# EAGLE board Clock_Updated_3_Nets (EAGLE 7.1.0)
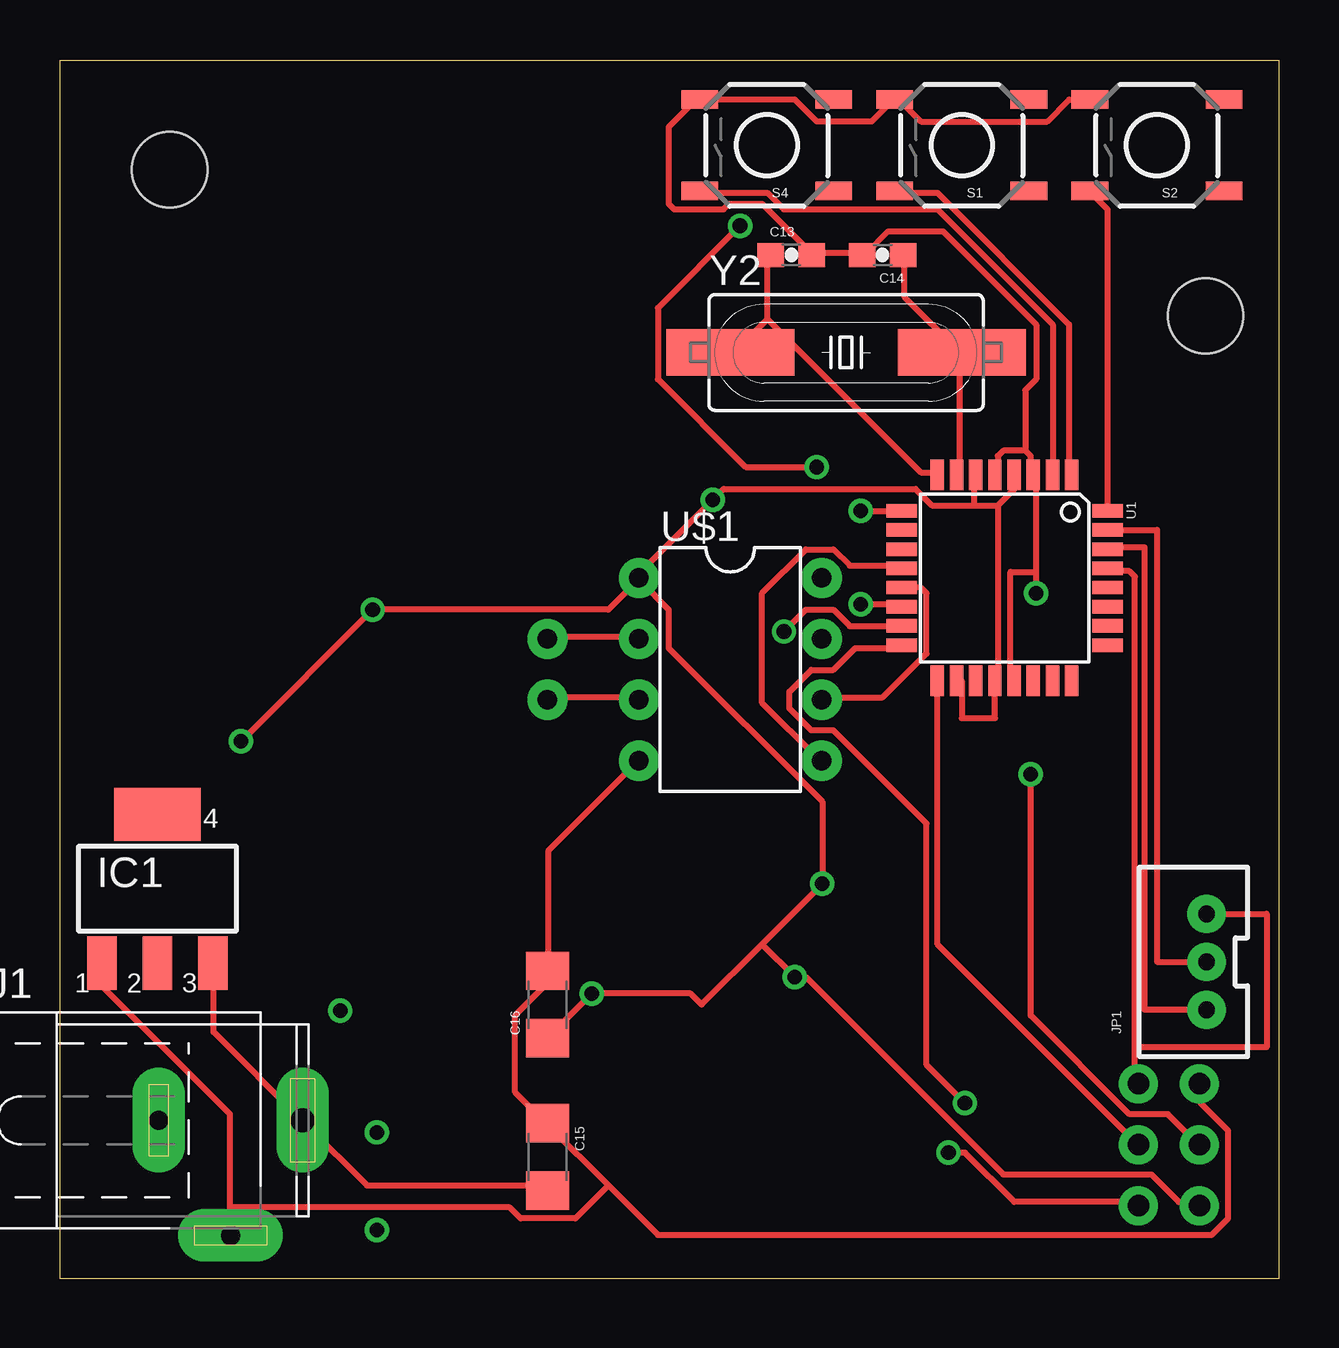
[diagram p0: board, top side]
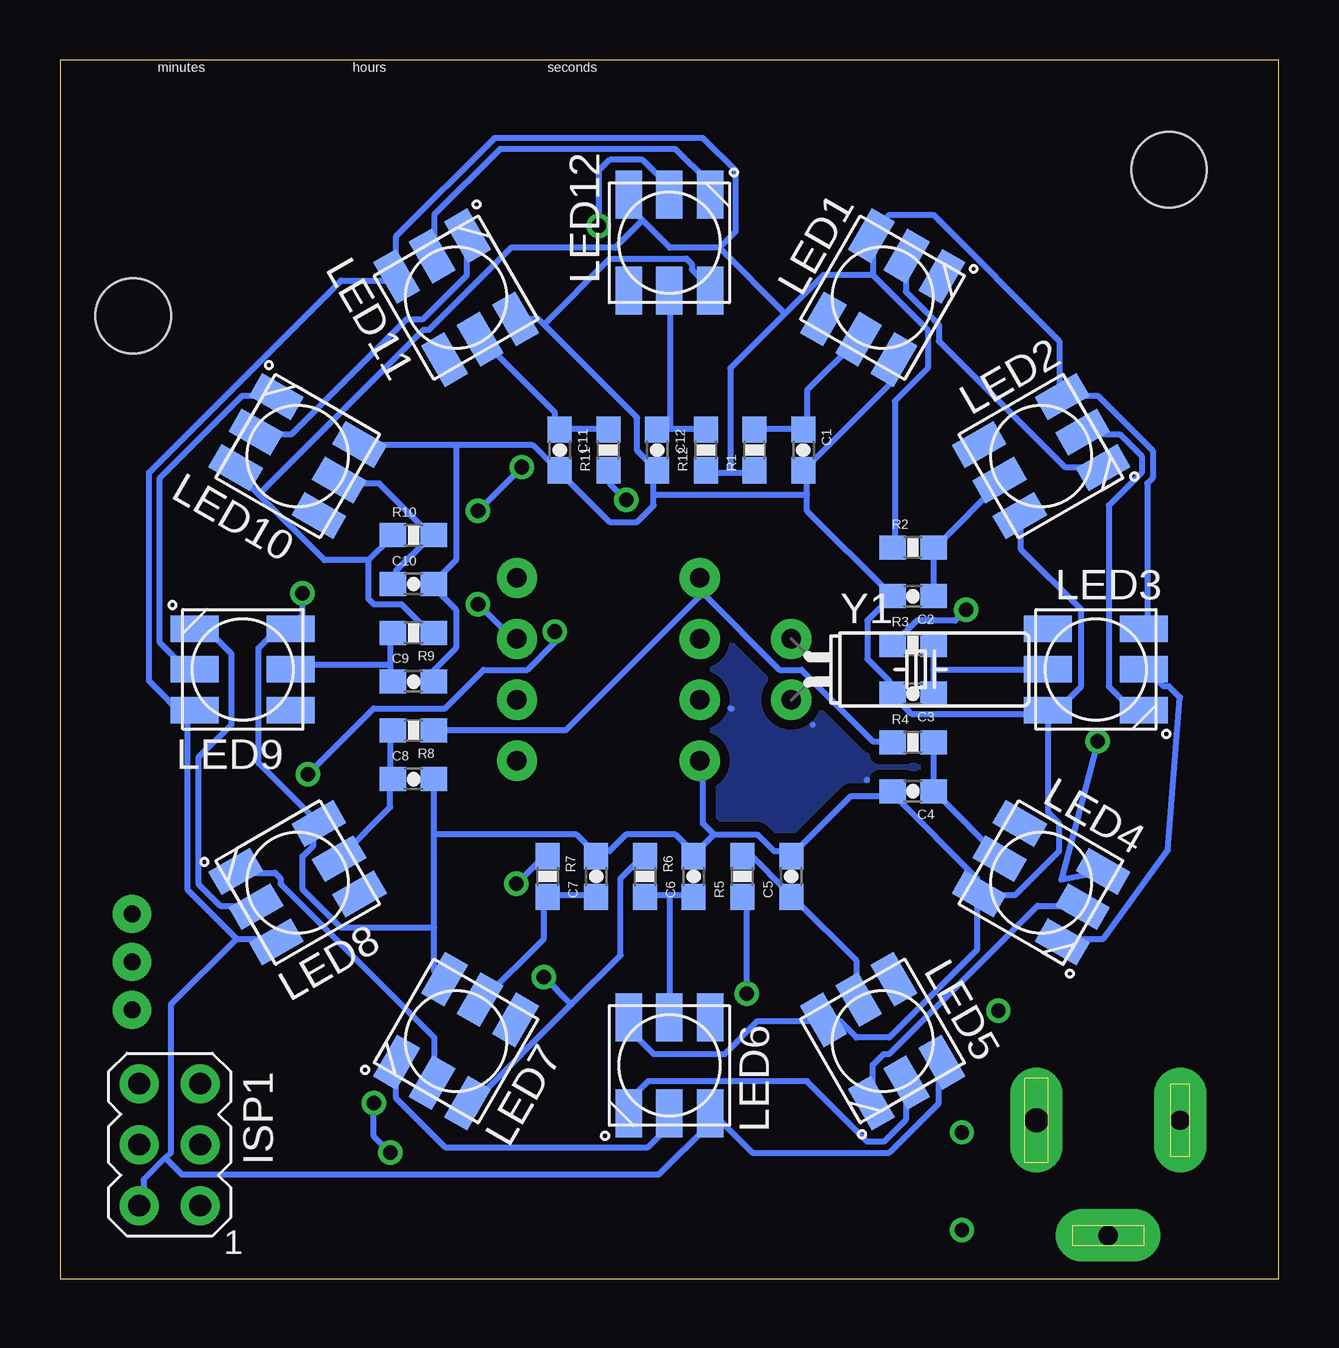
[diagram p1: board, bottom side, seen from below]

Size 50.8 x 50.8 mm. Coordinates in mm from the lower left corner, seen from the top.
Outline: 50.8,0 0,0 0,50.8 50.8,50.8 50.8,0
Copper layers (1*16): Top 0.035mm / dielectric 1.5mm / Bottom 0.035mm
Design rules "default": minimum track width 10mil, minimum drill 24mil, track to track 8mil, track to pad 8mil, pad to pad 8mil, via to via 8mil, smd to smd 8mil, copper to edge 40mil, drill to drill 8mil, minimum pad ring 10mil, minimum via ring 8mil, stop-mask expansion 4mil, vias tented up to drill 0mil, thermal gap 10mil
Holes 3.14 mm at 4.57,46.23 47.75,40.13

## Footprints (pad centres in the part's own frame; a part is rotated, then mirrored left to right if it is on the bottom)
0603-CAP = smd 1.1 x 1: 1 -0.85,0; 2 0.85,0
1206 = smd 1.6 x 1.8: 1 -1.4,0; 2 1.4,0
SOT223 = smd 1.219 x 2.235: 1 -2.311,-3.099; 2 0,-3.099; 3 2.311,-3.099 | smd 3.6 x 2.2: 4 0,3.099
AVRISP = drill 0.9 pad 1.626: 1 -1.27,2.54; 2 1.27,2.54; 3 -1.27,0; 4 1.27,0; 5 -1.27,-2.54; 6 1.27,-2.54
SPC4077 = drill 0.8 pad 2.184 long: 1 -3,0; 2 0,-4.8 | drill 1 pad 2.184 long: 3 3,0
JST-3-PTH-VERT = drill 0.7 pad 1.6: 1 -2,-0.55; 2 0,-0.55; 3 2,-0.55
WS2812 = smd 2 x 1.1: DI 2,0; DO 2,-1.7; LEDVDD -2,0; NC -2,1.7; VDD 2,1.7; VSS -2,-1.7
0603-RES = smd 1.1 x 1: 1 -0.85,0; 2 0.85,0
TACTILE-SWITCH-SMD = smd 1.524 x 0.762: 1 -2.794,1.905; 2 2.794,1.905; 3 -2.794,-1.905; 4 2.794,-1.905
TQFP32-08 = smd 1.27 x 0.559: 1 -4.293,2.8; 2 -4.293,2; 3 -4.293,1.2; 4 -4.293,0.4; 5 -4.293,-0.4; 6 -4.293,-1.2; 7 -4.293,-2; 8 -4.293,-2.8; 17 4.293,-2.8; 18 4.293,-2; 19 4.293,-1.2; 20 4.293,-0.4; 21 4.293,0.4; 22 4.293,1.2; 23 4.293,2; 24 4.293,2.8 | smd 0.559 x 1.27: 9 -2.8,-4.293; 10 -2,-4.293; 11 -1.2,-4.293; 12 -0.4,-4.293; 13 0.4,-4.293; 14 1.2,-4.293; 15 2,-4.293; 16 2.8,-4.293; 25 2.8,4.293; 26 2,4.293; 27 1.2,4.293; 28 0.4,4.293; 29 -0.4,4.293; 30 -1.2,4.293; 31 -2,4.293; 32 -2.8,4.293
DIL08-ROUND = drill 0.813 pad 1.676: 1 -3.81,-3.81; 2 -1.27,-3.81; 3 1.27,-3.81; 4 3.81,-3.81; 5 3.81,3.81; 6 1.27,3.81; 7 -1.27,3.81; 8 -3.81,3.81
TC38H = drill 0.813 pad 1.676: 1 -1.27,0; 2 1.27,0
HC49UP = smd 5.334 x 1.93: 1 -4.826,0; 2 4.826,0

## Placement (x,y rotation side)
C1  0.1uF  [0603-CAP]  19.81,34.54 270 bottom
C2  0.1uF  [0603-CAP]  15.24,28.45 180 bottom
C3  0.1uF  [0603-CAP]  15.24,24.38 180 bottom
C4  0.1uF  [0603-CAP]  15.24,20.32 180 bottom
C5  0.1uF  [0603-CAP]  20.32,16.76 90 bottom
C6  0.1uF  [0603-CAP]  24.38,16.76 90 bottom
C7  0.1uF  [0603-CAP]  28.45,16.76 90 bottom
C8  0.1uF  [0603-CAP]  36.07,20.83 0 bottom
C9  0.1uF  [0603-CAP]  36.07,24.89 0 bottom
C10  0.1uF  [0603-CAP]  36.07,28.96 0 bottom
C11  0.1uF  [0603-CAP]  29.97,34.54 270 bottom
C12  0.1uF  [0603-CAP]  25.91,34.54 270 bottom
C13  22pF  [0603-CAP]  30.48,42.67 0 top
C14  22pF  [0603-CAP]  34.29,42.67 180 top
C15  10uF  [1206]  20.32,5.08 270 top
C16  10uF  [1206]  20.32,11.43 90 top
IC1  317EMP  [SOT223]  4.06,16.26 0 top
ISP1  AVRISP-6  [AVRISP]  46.23,5.59 180 bottom
J1  [SPC4077]  7.11,6.6 0 top
JP1  [JST-3-PTH-VERT]  47.24,13.21 90 top
LED1  WS2812  [WS2812]  16.51,40.89 60 bottom
LED2  WS2812  [WS2812]  9.91,34.29 30 bottom
LED3  WS2812  [WS2812]  7.62,25.4 0 bottom
LED4  WS2812  [WS2812]  9.91,16.51 330 bottom
LED5  WS2812  [WS2812]  16.51,9.91 300 bottom
LED6  WS2812  [WS2812]  25.4,8.89 270 bottom
LED7  WS2812  [WS2812]  34.29,9.91 240 bottom
LED8  WS2812  [WS2812]  40.89,16.51 210 bottom
LED9  WS2812  [WS2812]  43.18,25.4 180 bottom
LED10  WS2812  [WS2812]  40.89,34.29 150 bottom
LED11  WS2812  [WS2812]  34.29,40.89 120 bottom
LED12  WS2812  [WS2812]  25.4,43.18 90 bottom
R1  180  [0603-RES]  21.84,34.54 90 bottom
R2  180  [0603-RES]  15.24,30.48 0 bottom
R3  180  [0603-RES]  15.24,26.42 0 bottom
R4  180  [0603-RES]  15.24,22.35 0 bottom
R5  180  [0603-RES]  22.35,16.76 90 bottom
R6  180  [0603-RES]  26.42,16.76 270 bottom
R7  180  [0603-RES]  30.48,16.76 270 bottom
R8  180  [0603-RES]  36.07,22.86 180 bottom
R9  180  [0603-RES]  36.07,26.92 180 bottom
R10  180  [0603-RES]  36.07,30.99 0 bottom
R11  180  [0603-RES]  27.94,34.54 90 bottom
R12  180  [0603-RES]  23.88,34.54 90 bottom
S1  TAC_SWITCHSMD  [TACTILE-SWITCH-SMD]  37.59,47.24 180 top
S2  TAC_SWITCHSMD  [TACTILE-SWITCH-SMD]  45.72,47.24 180 top
S4  TAC_SWITCHSMD  [TACTILE-SWITCH-SMD]  29.46,47.24 180 top
U1  ATMEGA328P  [TQFP32-08]  39.37,29.21 270 top
U$1  DS1302  [DIL08-ROUND]  27.94,25.4 270 top
Y1  [TC38H]  20.32,25.4 270 bottom
Y2  [HC49UP]  32.77,38.61 0 top

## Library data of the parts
C1-C12 = SparkFun-Capacitors; PROD_ID: CAP-00810
C13 C14 = SparkFun-Capacitors; PROD_ID: CAP-07876
C15 C16 = SparkFun-Capacitors; PROD_ID: CAP-10057
IC1 = linear
ISP1 LED1-LED12 U$1 = adafruit
J1 = con-jack; OC_FARNELL: unknown; OC_NEWARK: unknown
JP1 = SparkFun-Connectors
R1-R12 = SparkFun-Resistors; PROD_ID: RES-08788
S1 S2 S4 = SparkFun-Electromechanical; PROD_ID: SWCH-08247
U1 = SparkFun-DigitalIC; PROD_ID: IC-09069
Y1 Y2 = SparkFun-FreqCtrl

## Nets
GND: C1.2 C2.2 C3.2 C4.2 C5.2 C6.2 C7.2 C8.2 C9.2 C10.2 C11.2 C12.2 C13.2 C14.2 C15.1 C16.2 IC1.1 ISP1.6 J1.2 LED1.VSS LED2.VSS LED3.VSS LED4.VSS LED5.VSS LED6.VSS LED7.VSS LED8.VSS LED9.VSS LED10.VSS LED11.VSS LED12.VSS S1.4 S2.4 S4.4 U1.3 U1.5 U1.21 U$1.4
N$1: ISP1.4 U1.15
N$2: ISP1.1 U1.16
N$3: JP1.1 U1.30
N$4: S2.2 U1.32
N$5: U$1.3 Y1.2
N$6: U$1.2 Y1.1
N$7: C1.1 LED1.LEDVDD R1.2
N$8: C2.1 LED2.LEDVDD R2.2
N$9: LED1.DI LED2.DO
N$10: C3.1 LED3.LEDVDD R3.2
N$11: C4.1 LED4.LEDVDD R4.2
N$12: LED3.DI LED4.DO
N$13: C5.1 LED5.LEDVDD R5.2
N$14: C6.1 LED6.LEDVDD R6.2
N$15: LED5.DI LED6.DO
N$16: C7.1 LED7.LEDVDD R7.2
N$17: C8.1 LED8.LEDVDD R8.2
N$18: LED7.DI LED8.DO
N$19: C9.1 LED9.LEDVDD R9.2
N$20: C10.1 LED10.LEDVDD R10.2
N$21: LED9.DI LED10.DO
N$22: C11.1 LED11.LEDVDD R11.2
N$23: C12.1 LED12.LEDVDD R12.2
N$24: LED11.DI LED12.DO
N$25: LED4.DI LED5.DO
N$26: LED8.DI LED9.DO
N$27: JP1.2 U1.31
N$30: S1.2 U1.1
N$31: U1.13 U$1.6
N$32: U1.12 U$1.5
N$33: U1.14 U$1.7
N$34: ISP1.3 U1.17
N$36: ISP1.5 JP1.3 U1.29
N$37: S4.2 U1.2
N$38: C13.1 U1.8 Y2.1
N$40: LED2.DI LED3.DO
N$41: LED6.DI LED7.DO
N$42: LED10.DI LED11.DO
N$43: LED12.DI U1.9
N$44: C14.1 U1.7 Y2.2
N$45: C15.2 IC1.3 J1.3
VBAT: U$1.8
VCC: C16.1 ISP1.2 LED1.VDD LED2.VDD LED3.VDD LED4.VDD LED5.VDD LED6.VDD LED7.VDD LED8.VDD LED9.VDD LED10.VDD LED11.VDD LED12.VDD R1.1 R2.1 R3.1 R4.1 R5.1 R6.1 R7.1 R8.1 R9.1 R10.1 R11.1 R12.1 U1.4 U1.6 U1.18 U1.20 U$1.1

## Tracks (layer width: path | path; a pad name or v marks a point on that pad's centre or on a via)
GND  (via drill 0.61)
  Top 0.254: 40.23,34.52 39.32,34.52 39.09,34.29 39.09,33.6 U1.5 | 40.23,34.52 40.46,34.29 40.46,33.6 U1.3 40.69,33.38 40.69,29.46 | S2.4 42.06,49.15 41.15,48.23 35.89,48.23 34.98,49.15 S1.4 34.75,49.15 33.83,48.23 31.55,48.23 30.63,49.15 S4.4 26.52,49.15 25.38,48.01 25.38,44.81 25.6,44.58 27.66,44.58 27.89,44.81 29.26,44.81 31.32,42.75 C13.2 31.55,42.75 33.38,42.75 C14.2 33.6,42.75 34.52,43.66 36.8,43.66 40.69,39.78 40.69,37.49 40.23,37.03 40.23,34.52 | v40.69,28.57 40.69,29.46 | U$1.4 24,21.49 20.34,17.83 20.34,13.03 C16.2 20.12,12.8 20.12,12.12 18.97,10.97 18.97,7.77 20.12,6.63 C15.1 20.34,6.4 22.86,3.89 | U1.21 39.62,24.92 39.62,29.46 40.69,29.46 | 7.09,2.97 7.09,1.83 J1.2 | 7.09,2.97 7.09,6.86 1.83,12.12 1.83,13.03 IC1.1 | 22.86,3.89 24.92,1.83 48.01,1.83 48.69,2.52 48.69,6.17 47.55,7.32 47.55,8 ISP1.6 | 7.09,2.97 18.75,2.97 19.2,2.52 21.49,2.52 22.86,3.89
  Bottom 0.254: LED1.VSS 16.23,38.18 16.23,37.26 19.66,33.83 C1.2 19.66,33.6 19.66,32.69 | LED3.VSS 9.83,23.55 15.32,23.55 16,24.23 C3.2 16.23,24.46 16.23,24.92 17.14,25.83 17.14,27.43 16.23,28.35 C2.2 16.23,28.57 19.66,32 19.66,32.69 | LED2.VSS 10.74,31.77 10.74,30.4 8.23,27.89 8.23,24.69 9.14,23.77 9.6,23.77 LED3.VSS | C9.2 35.2,24.92 35.2,25.38 34.29,26.29 34.29,27.89 35.2,28.8 C10.2 35.2,29.03 34.29,29.95 34.29,34.75 | 26.06,32.69 26.06,32.23 26.75,31.55 27.89,31.55 29.95,33.6 C11.2 30.18,33.83 31.09,34.75 34.29,34.75 | 26.06,32.69 26.06,33.6 C12.2 26.06,33.83 26.75,34.52 26.75,35.89 30.63,39.78 | 34.29,34.75 38.18,34.75 LED10.VSS | 30.63,39.78 30.86,40.01 31.77,40.01 LED11.VSS | 30.63,39.78 27.89,42.52 24.69,42.52 24.46,42.29 24.46,42.06 23.77,41.38 LED12.VSS | 26.06,32.69 19.66,32.69 | 35.2,14.63 35.2,12.8 34.98,12.57 LED7.VSS | 35.2,14.63 35.2,18.52 | 35.2,18.52 35.2,20.8 C8.2 | 35.2,14.63 39.09,14.63 40.69,16.23 40.69,17.6 40.23,18.06 40.23,18.97 LED8.VSS 40.23,19.2 42.52,21.49 42.52,26.29 41.83,26.98 41.38,26.98 LED9.VSS 41.15,27.2 40.69,27.66 v40.69,28.57 | LED6.VSS 26.98,10.74 26.98,10.29 26.06,9.37 23.09,9.37 21.72,10.74 19.2,10.74 LED5.VSS 18.97,10.74 18.29,10.74 17.6,10.06 16.23,10.06 12.57,13.72 12.57,16 LED4.VSS | 23.55,18.52 21.72,18.52 21.03,17.83 20.34,17.83 C5.2 20.12,17.83 17.83,20.12 16.23,20.12 C4.2 16,20.12 12.57,16.69 12.57,16.23 LED4.VSS | 23.55,18.52 24.23,17.83 C6.2 24.46,17.83 25.15,18.52 27.2,18.52 27.89,17.83 28.35,17.83 C7.2 28.57,17.83 29.26,18.52 35.2,18.52 | 23.55,18.52 24,18.97 24,21.49 U$1.4 | LED3.VSS 9.6,23.55 9.6,19.43 9.14,18.97 9.14,17.83 10.97,16 12.34,16 LED4.VSS
N$1  (via drill 0.61)
  Top 0.254: v30.18,26.98 31.09,27.89 32.23,27.89 32.92,27.2 34.98,27.2 U1.15 | v40.46,21.03 40.46,10.97 44.58,6.86 46.18,6.86 47.32,5.71 ISP1.4
  Bottom 0.254: v30.18,26.98 30.18,26.52 31.32,25.38 33.15,25.38 34.75,23.77 37.72,23.77 v40.46,21.03
N$2  (via drill 0.61)
  Top 0.254: v37.72,7.32 36.12,8.91 36.12,18.97 32.23,22.86 31.32,22.86 30.4,23.77 30.4,24.46 31.32,25.38 32.23,25.38 33.15,26.29 34.98,26.29 U1.16 | v37.03,5.26 37.72,5.26 39.78,3.2 44.81,3.2 ISP1.1
  Bottom 0.254: v37.72,7.32 37.72,5.94 v37.03,5.26
N$3
  Top 0.254: JP1.1 45.21,11.21 45.21,30.48 43.66,30.48 U1.30
N$4
  Top 0.254: U1.32 43.66,44.58 42.98,45.26 S2.2
N$5
  Top 0.254: Y1.2 20.34,24.23 24,24.23 U$1.3
N$6
  Top 0.254: Y1.1 20.34,26.75 24,26.75 U$1.2
N$7
  Bottom 0.254: R1.2 21.72,35.43 19.89,35.43 C1.1 19.66,35.43 19.66,37.03 17.6,39.09 LED1.LEDVDD
N$8
  Bottom 0.254: C2.1 14.4,28.57 14.4,30.4 R2.2 14.17,30.63 11.66,33.15 LED2.LEDVDD
N$9
  Bottom 0.254: LED2.DO 7.54,33.83 8.91,33.83 14.17,39.09 14.17,39.78 15.54,41.15 15.54,42.52 LED1.DI
N$10
  Bottom 0.254: 14.4,25.38 14.4,26.29 R3.2 | 14.4,25.38 14.4,24.46 C3.1 | 14.4,25.38 9.83,25.38 LED3.LEDVDD
N$11
  Bottom 0.254: R4.2 14.4,22.17 14.4,20.34 C4.1 14.17,20.12 11.66,17.6 LED4.LEDVDD
N$12
  Bottom 0.254: LED3.DI 5.49,25.38 4.8,24.69 4.57,24.69 4.12,24.23 4.62,17.88 7.32,14.17 8.91,14.17 LED4.DO
N$13
  Bottom 0.254: R5.2 22.17,17.83 20.34,16 C5.1 20.12,15.77 17.6,13.26 17.6,11.66 LED5.LEDVDD
N$14
  Bottom 0.254: 25.38,16 26.29,16 R6.2 | 25.38,16 24.46,16 C6.1 | 25.38,16 25.38,10.97 LED6.LEDVDD
N$15
  Bottom 0.254: LED6.DO 26.98,7.09 26.98,7.54 26.29,8.23 19.66,8.23 17.14,5.71 16.46,5.71 15.54,6.63 15.54,8 LED5.DI
N$16
  Bottom 0.254: C7.1 28.57,16 30.4,16 R7.2 30.63,15.77 30.63,14.17 33.15,11.66 LED7.LEDVDD
N$17
  Bottom 0.254: R8.2 37.03,22.86 37.03,21.03 C8.1 37.03,20.8 37.03,19.66 39.09,17.6 LED8.LEDVDD
N$18
  Bottom 0.254: LED7.DI 35.2,8.23 35.2,10.06 41.6,16.46 41.6,16.69 41.83,16.92 43.43,16.92 LED8.DO
N$19
  Bottom 0.254: 37.03,25.6 37.03,26.75 R9.2 | 37.03,25.6 37.03,24.92 C9.1 | 37.03,25.6 41.15,25.6 LED9.LEDVDD
N$20
  Bottom 0.254: C10.1 36.8,29.03 36.8,29.49 35.43,30.86 R10.2 35.43,31.09 37.49,33.15 39.09,33.15 LED10.LEDVDD
N$21
  Bottom 0.254: LED10.DO 41.83,36.8 43.2,36.8 46.63,33.38 46.63,26.52 45.72,25.6 45.26,25.6 LED9.DI
N$22
  Bottom 0.254: R11.2 28.12,35.43 29.95,35.43 C11.1 30.18,35.43 30.18,36.12 33.15,39.09 LED11.LEDVDD
N$23
  Bottom 0.254: 25.38,35.43 25.83,35.43 C12.1 | 25.38,35.43 24,35.43 R12.2 | 25.38,35.43 25.38,41.15 LED12.LEDVDD
N$24
  Bottom 0.254: LED11.DI 35.2,42.75 35.2,44.35 32.46,47.09 25.15,47.09 23.77,45.72 23.77,45.26 LED12.DO
N$25
  Bottom 0.254: LED5.DO 16.92,7.54 16.92,8.91 16.46,9.37 16.23,9.37 10.06,15.54 8.23,15.54 LED4.DI
N$26
  Bottom 0.254: LED8.DI 42.75,15.54 44.12,15.54 45.03,16.46 45.03,21.72 43.66,23.09 43.66,26.06 44.58,26.98 45.03,26.98 LED9.DO
N$27
  Top 0.254: U1.31 45.72,31.21 45.72,13.21 JP1.2
N$28
  Bottom 0.254: 22.86,23.77 22.8,23.75 | 17.14,20.8 17.17,20.78 | 19.43,23.09 19.43,23.08
  pour Bottom (isolate 0.406): 0.51,50.29 50.29,50.29 50.8,50.29 50.8,0 0,0 0,50.29
N$29  (via drill 0.6)
  other vias: 13.21,2.03
N$30
  Top 0.254: U1.1 42.06,33.6 42.06,39.78 36.58,45.26 34.98,45.26 S1.2
N$31
  Top 0.254: U1.13 35.2,28.8 35.89,28.8 36.12,28.57 36.12,26.06 34.29,24.23 31.77,24.23 U$1.6
N$32
  Top 0.254: U1.12 34.98,29.72 32.92,29.72 32.23,30.4 31.09,30.4 29.26,28.57 29.26,24 31.55,21.72 U$1.5
N$33  (via drill 0.61)
  Top 0.254: v33.38,28.12 34.98,28.12 U1.14
  Bottom 0.254: v33.38,28.12 31.77,26.52 U$1.7
N$34
  Top 0.254: U1.17 36.58,13.95 44.81,5.71 ISP1.3
N$35  (via drill 0.6)
  other vias: 13.21,6.1
N$36
  Top 0.254: 44.81,9.65 44.81,8.23 ISP1.5 | 44.81,9.65 44.81,29.26 44.58,29.49 43.66,29.49 U1.29 | JP1.3 50.29,15.21 50.29,9.65 44.81,9.65
N$37
  Top 0.254: U1.2 41.38,33.6 41.38,39.78 36.58,44.58 30.18,44.58 29.49,45.26 26.75,45.26 S4.2
N$38
  Top 0.254: 29.49,40.01 29.49,42.52 C13.1 | 29.49,40.01 28.12,38.63 Y2.1 | 29.49,40.01 35.89,33.6 36.35,33.6 U1.8
N$39  (via drill 0.6)
  other vias: 11.68,11.18
N$40
  Bottom 0.254: LED3.DO 5.71,23.77 6.17,23.77 7.09,24.69 7.09,32.23 5.71,33.6 5.71,34.29 6.63,35.2 8,35.2 LED2.DI
N$41
  Bottom 0.254: LED6.DI 25.6,6.86 25.6,6.17 26.29,5.49 34.75,5.49 36.8,7.54 36.8,8.91 LED7.DO
N$42
  Bottom 0.254: LED11.DO 33.83,43.43 33.83,41.83 35.66,40.01 36.35,40.01 41.15,35.2 42.52,35.2 LED10.DI
N$43  (via drill 0.61)
  Top 0.254: v33.38,32 34.98,32 U1.9 | v31.55,33.83 28.57,33.83 24.92,37.49 24.92,40.46 v28.35,43.89
  Bottom 0.254: v31.55,33.83 v33.38,32 | v28.35,43.89 28.35,46.18 27.89,46.63 26.52,46.63 25.6,45.72 25.6,45.26 LED12.DI
N$44
  Top 0.254: C14.1 35.2,42.52 35.2,40.92 37.49,38.63 Y2.2 37.49,38.41 37.49,33.6 U1.7
N$45
  Top 0.254: C15.2 20.12,3.89 12.8,3.89 10.29,6.4 J1.3 10.06,6.63 6.4,10.29 6.4,13.03 IC1.3
VCC  (via drill 0.61)
  Top 0.254: C16.1 20.34,10.06 v22.17,11.89 26.29,11.89 26.75,11.43 29.26,13.95 | 29.26,13.95 v31.77,16.46 31.77,19.89 25.38,26.29 25.38,27.89 24.23,29.03 U$1.1 | 29.26,13.95 v30.63,12.57 31.09,12.57 39.32,4.34 45.49,4.34 46.63,3.2 47.32,3.2 ISP1.2 | 39.09,32.23 39.09,24.92 U1.20 38.97,23.37 37.59,23.37 37.59,24.92 U1.18 | 39.09,32.23 39.78,32.92 39.78,33.38 U1.4 | U$1.1 24,29.03 22.86,27.89 v13.03,27.89 v7.54,22.4 | U$1.1 24,29.26 v27.2,32.46 27.66,32.92 35.66,32.92 36.35,32.23 38.1,32.23 | 38.1,32.23 39.09,32.23 | U1.6 38.1,33.5 38.1,32.23
  Bottom 0.254: 37.95,29.95 37.95,28.35 37.72,28.12 36.58,28.12 35.43,26.98 R9.1 | 37.95,29.95 37.03,30.86 R10.1 | 42.52,32.69 39.78,29.95 37.95,29.95 | 42.52,32.69 43.43,33.6 LED10.VDD | LED3.VDD 5.49,27.2 5.49,33.15 5.26,33.38 5.26,34.52 7.54,36.8 8.91,36.8 LED2.VDD 9.14,36.8 9.14,39.09 14.4,44.35 16.23,44.35 16.92,43.66 LED1.VDD 16.92,43.43 16.92,41.83 | 22.86,33.6 23.77,33.6 R12.1 | 22.86,33.6 21.95,33.6 R1.1 | 16.92,41.83 14.63,39.55 14.63,37.95 16,36.58 16,30.63 R2.1 | 22.86,33.6 22.86,37.95 20.57,40.23 | 20.57,40.23 18.97,41.83 16.92,41.83 | 26.52,44.12 25.38,42.98 23.32,42.98 | 26.52,44.12 26.98,44.58 26.98,45.03 LED12.VDD | 20.57,40.23 23.32,42.98 | 23.32,42.98 22.63,43.66 22.63,46.18 24,47.55 32.69,47.55 36.8,43.43 36.8,41.83 LED11.VDD 36.8,41.6 39.09,41.6 47.09,33.6 47.09,24.92 45.49,23.32 | 42.52,32.69 35.66,39.55 35.43,39.55 32,42.98 27.66,42.98 26.52,44.12 | LED5.VDD 14.17,8.91 14.17,7.32 16.23,5.26 21.95,5.26 23.55,6.86 LED6.VDD 23.77,6.86 23.77,6.4 25.83,4.34 45.72,4.34 46.41,5.03 | 43.43,14.17 41.83,14.17 LED8.VDD | 43.43,14.17 45.49,16.23 45.49,23.32 | 45.49,23.32 45.26,23.55 LED9.VDD 45.49,23.32 | 46.41,5.03 46.18,5.26 46.18,11.43 43.43,14.17 | 46.41,5.03 47.32,4.12 47.32,3.2 ISP1.2 | 29.49,11.43 33.6,7.32 LED7.VDD | 29.49,11.43 27.43,13.49 27.43,16.69 26.52,17.6 R6.1 | v22.17,11.89 22.17,15.77 R5.1 | v31.77,16.46 30.63,17.6 R7.1 | v30.63,12.57 29.49,11.43 | 24,28.57 20.8,25.38 19.89,25.38 16.92,22.4 16.23,22.4 R4.1 | 24,28.57 24,29.03 U$1.1 24,28.57 | v13.03,27.89 13.49,27.43 15.09,27.43 16,26.52 R3.1 | R8.1 29.72,22.86 24,28.57 | v27.2,32.46 27.89,33.15 27.89,33.6 R11.1
  Bottom 0.254: v7.54,22.4 9.07,16.64 LED4.VDD

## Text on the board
bPlace: seconds | hours | minutes

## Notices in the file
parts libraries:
SparkFun-Capacitors: Licensing: Creative Commons ShareAlike 4.0 International - https://creativecommons.org/licenses/by-sa/4.0
